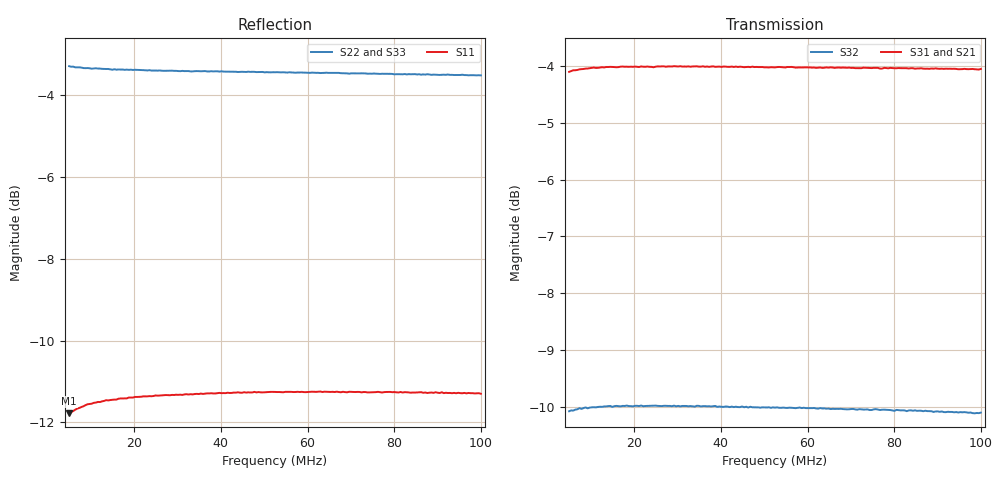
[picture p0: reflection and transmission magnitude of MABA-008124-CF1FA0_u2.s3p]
#	MHz	S	dB	R	75
!FREQ	R1	I1	R2	I2	R3	I3
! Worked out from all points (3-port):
!   201 points, 5 MHz to 100 MHz, reference 75 ohm
!   strongest paths, dB at 5 MHz, 28.75 MHz, 52.5 MHz, 76.25 MHz, 100 MHz:
!     S31: -4.1, -4.0, -4.0, -4.0, -4.1
!     S21: -4.1, -4.0, -4.0, -4.0, -4.0
!     S32: -10.1, -10.0, -10.0, -10.1, -10.1
!   lowest |S11| = -11.8 dB at 5 MHz (marker M1), VSWR 1.69, Z = 124 + j15.3 ohm
!   |S11| at or under -10 dB: start of sweep to end of sweep
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5  -11.78 12.9  -4.11 -177.9  -4.10 2.2
   -4.10 -177.9  -3.30 178.2  -10.08 -177.7
   -4.10 2.2  -10.08 -177.7  -3.28 178.3
7.375  -11.65 9.4  -4.07 -178.7  -4.06 1.3
       -4.07 -178.8  -3.33 178.2  -10.04 -178.6
       -4.06 1.3  -10.02 -178.6  -3.31 178.3
9.75  -11.55 7.3  -4.05 -179.3  -4.04 0.7
      -4.05 -179.4  -3.35 178.1  -10.01 -179.2
      -4.04 0.7  -10.02 -179.2  -3.32 178.3
12.6  -11.49 5.8  -4.03 -179.8  -4.02 0.2
      -4.03 -180.0  -3.36 178.0  -10.00 -179.6
      -4.02 0.2  -10.00 -179.7  -3.34 178.2
16.875  -11.42 4.3  -4.02 179.5  -4.01 -0.4
        -4.02 179.4  -3.38 177.7  -9.99 179.7
        -4.01 -0.4  -9.99 179.8  -3.35 177.9
30.65  -11.32 1.7  -4.01 178.0  -4.00 -1.9
       -4.02 177.7  -3.42 176.6  -9.98 178.3
       -4.00 -1.9  -9.99 178.3  -3.38 176.9
52.5  -11.26 -0.6  -4.03 176.0  -4.02 -3.9
      -4.03 175.5  -3.45 174.8  -10.01 176.5
      -4.02 -3.9  -10.01 176.5  -3.40 175.2
63.9  -11.25 -1.6  -4.03 175.0  -4.03 -4.9
      -4.04 174.5  -3.46 173.7  -10.03 175.5
      -4.03 -4.9  -10.03 175.6  -3.41 174.2
90.975  -11.26 -3.4  -4.02 172.7  -4.05 -7.1
        -4.04 172.0  -3.51 171.6  -10.08 173.5
        -4.05 -7.1  -10.08 173.5  -3.41 172.1
100  -11.30 -4.0  -4.01 171.9  -4.05 -7.9
     -4.04 171.2  -3.52 170.8  -10.10 172.9
     -4.05 -7.9  -10.10 172.9  -3.42 171.3
